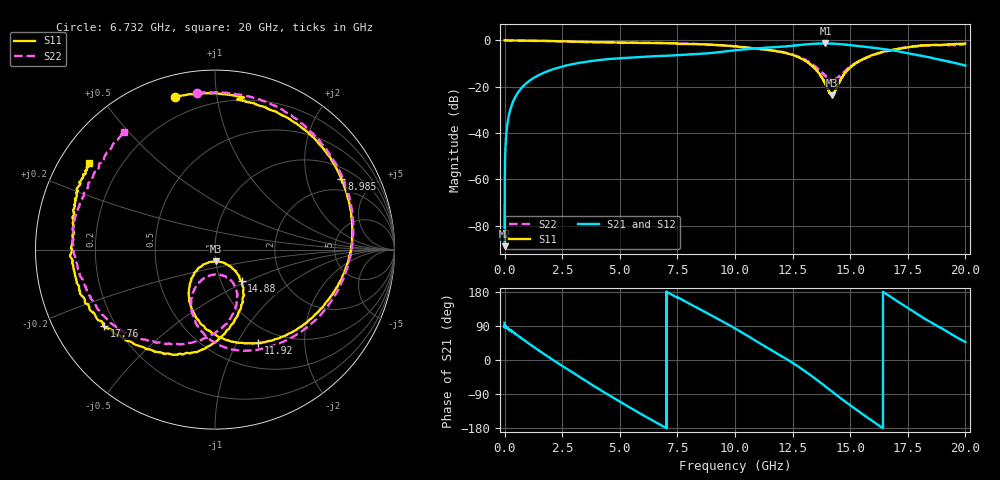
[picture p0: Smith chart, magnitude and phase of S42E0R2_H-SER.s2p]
!{S42E0R2}
!Johanson Technology Inc.
!www.johansontechnology.com
!Test Board Conditions:
!Substrate Type  RO4350B
!Substrate Thickness  50 mil
!Substrate Dk  3.66
!TL Type: GCPW
!TL Trace Width  60 mil
!TL Gap  10 mil
!Electrode orientation  Horizontal
!DUT TOPOLOGY	SERIES
!Mounting Pad LxW  14x55 mil
! Created Wed Nov 25 20:15:03 2020
# khz S ma R 50
! 2 Port Network Data from SP1.SP block
! freq  magS11  angS11  magS21  angS21  magS12  angS12  magS22  angS22
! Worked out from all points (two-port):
!   20001 points, 300 kHz to 20 GHz, reference 50 ohm
!   highest |S21| = -1.27 dB at 13.93 GHz (marker M1); lowest = -88.8 dB at 300 kHz (marker M2)
!   |S21| within 3 dB of the highest: 9.984673 GHz to 9.994237 GHz (9.564 MHz wide, 0.0957 % of centre); 9.994 GHz to 16.82 GHz (6.827 GHz wide, 50.9 % of centre)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
!   lowest |S11| = -23.7 dB at 14.21 GHz (marker M3), VSWR 1.14, Z = 49.9 - j6.51 ohm
!   |S11| at or under -10 dB: 13.23 GHz to 15.22 GHz (1.983 GHz wide, 13.9 % of centre)
!   |S22| runs from -17.2 to 0.0 dB; largest |S21 - S12| = 0.019
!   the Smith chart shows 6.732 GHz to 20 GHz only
!   S11 on the Smith chart (normalised r, x): 6.732 GHz: 0.10, +0.77; 8.985 GHz: 1.44, +3.25; 11.92 GHz: 0.79, -1.23; 14.88 GHz: 1.25, -0.47; 17.76 GHz: 0.15, -0.30; 20 GHz: 0.09, +0.31
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300  0.9998 -0.3  3.624e-05 98.2  5.485e-05 -101.9  1 -0.4
103300  0.9992 -4.6  0.0135 85.0  0.01362 85.1  0.9999 -4.7
143300  0.999 -6.2  0.01877 83.2  0.01878 83.1  0.9992 -6.4
533300  0.9969 -23.6  0.06899 66.2  0.06924 66.2  0.9975 -24.3
1908300  0.975 -81.6  0.2209 7.9  0.2218 7.9  0.9708 -82.3
3334300  0.9331 -138.2  0.334 -47.7  0.3342 -47.8  0.9328 -136.4
4801300  0.9056 169.0  0.4064 -102.5  0.407 -102.8  0.9036 167.0
6667300  0.8788 106.9  0.4613 -167.8  0.4605 -168.1  0.8824 98.7
6732300  0.8788 104.8  0.4629 -170.0  0.4618 -170.3  0.8808 96.6
7875300  0.8378 68.2  0.4933 153.2  0.4898 153.4  0.8572 59.8
8985300  0.807 29.2  0.537 117.4  0.5391 117.8  0.8121 26.6
1.00003e7  0.7457 -4.4  0.6129 83.3  0.6116 83.5  0.7451 -7.0
1.19163e7  0.5727 -65.1  0.7279 14.1  0.7317 13.9  0.5781 -76.1
1.33343e7  0.2861 -120.9  0.8401 -42.8  0.8386 -42.9  0.3095 -115.2
1.39273e7  0.115 -128.2  0.8638 -70.0  0.8551 -69.7  0.1712 -110.7
1.42133e7  0.06502 -87.2  0.8552 -83.5  0.853 -83.2  0.1388 -89.9
1.48823e7  0.2301 -49.8  0.8055 -114.4  0.806 -114.3  0.2445 -61.5
1.57663e7  0.4414 -79.2  0.7174 -152.7  0.7209 -152.8  0.4342 -84.4
1.66673e7  0.6004 -106.0  0.6308 170.5  0.6165 170.5  0.5988 -119.2
1.77573e7  0.7519 -145.5  0.4982 127.4  0.509 128.0  0.7333 -155.8
1.88053e7  0.7976 176.8  0.3921 88.9  0.3921 88.5  0.8004 170.6
2e7  0.8554 145.6  0.2862 47.6  0.2884 48.5  0.8258 127.7
